PROGRAM MAIN

VAR CONSTANT
	// init pars for FB_CMA_SourcePaired, one dimensional signals with defined length
    cInitSourceVibration	: ST_MA_MultiArray_InitPars := (eTypeCode := eMA_TypeCode_LREAL, nDims := 1, aDimSizes := [cBufferLengthVib]);
	cInitSourcePosition		: ST_MA_MultiArray_InitPars := (eTypeCode := eMA_TypeCode_LREAL, nDims := 1, aDimSizes := [cBufferLengthPos]);	
END_VAR

VAR
	(* Properties of generated synthetic signals *)
	Amplitude			: ARRAY [0..9]  OF LREAL := [5, 8, 4, 7, 10, 9, 0, 0, 0, 0];
	Orders       		: ARRAY [0..9]  OF LREAL := [20, 50 , 90, 100, 120, 0, 0, 0, 0, 0];
	fbvib 				: FB_VibrationSource(Amplitude, Orders, cShaftPerimeter);
	aBufferVibration	: ARRAY[1..cOversamples] OF LREAL;  // vibration signal 
	aBufferPosition		: LREAL;                            // position signal
	
	(* Virtual axis control *)
	axis 				: AXIS_REF;
	fb_power 			: MC_POWER;
	fb_move 			: MC_MoveAbsolute;
	fb_reset 			: MC_Reset;
	
	(* axis control *)
	nstate 			: UDINT;
	nmovestate 		: UDINT;
	
	(* Sources and sinks *)
	fbSourceOrderSpec	: FB_CMA_SourcePaired :=(	stInitParsA := cInitSourceVibration, 
													stInitParsB := cInitSourcePosition,
													nOwnID := eID_SourcePaired, aDestIDs := [eID_OrderSpec], nResultBuffers := 4 );	// Initialize source buffers
	fbSourcePowerSpec	: FB_CMA_Source :=(	stInitPars := cInitSourceVibration, nOwnID := eID_Source, aDestIDs := [eID_PwrSpec], nResultBuffers := 4 );	// Initialize source buffers
	
	fbSinkOrderSpec		: FB_CMA_Sink := (nOwnID := eID_Sink_OrderSpec);
	fbSinkPowerSpec		: FB_CMA_Sink := (nOwnID := eID_Sink_PwrSpec);
	
	(* Spectrum results *)	
	aOrderSpecResult	: ARRAY[1..cFFTResult] OF LREAL;	// Copy of result
	aPowerSpecResult	: ARRAY[1..cFFTResult] OF LREAL;	// Copy of result
	
	(* Reset analysis chain *)
	bReset				: BOOL := FALSE;

	(* Helper *)
	i					: UDINT;
	{attribute 'BaseUnit' := '< AngularVelocity, 1, 0, None>'}
	fMotorspeed 			: LREAL;
	{attribute 'BaseUnit' := '< Angular, 1, 0, None>'}
	fMotorposition 		: LREAL;
	{attribute 'BaseUnit' := '< Angular, 1, 0, None>'}
	
	(* error monitoring *)
	fbErrHist			: FB_HRErrHist; // 
END_VAR

(* Axis control - Order spectrum specific code, see line 78ff*)
fb_power(Axis := axis);
fb_move(Axis := axis);
fb_reset(Axis := axis);
axis.ReadStatus();
CASE nstate OF 
	0: (* Reset axis *)
		fb_move.Execute := FALSE;
		fb_reset(Axis := axis, Execute := TRUE);
		fb_reset.Execute := TRUE;
		IF NOT fb_reset.Busy THEN
			nstate := 1;
		END_IF
		
	1:	(* Enable axis *)
		fb_reset.Execute := FALSE;
		fb_power.Enable := TRUE;
		fb_power.Enable_Positive := TRUE;
		fb_power.Enable_Negative := TRUE;
		IF axis.Status.ControlLoopClosed THEN
			nstate :=2;
		END_IF 
		
	2:	(* Run virtual axis *)	
		CASE nmovestate OF
			0:
				fb_reset.Execute := FALSE;;
				fb_move.Position := 10000;
				fb_move.Velocity := 20 *cShaftPerimeter;
				fb_move.BufferMode := MC_Buffered;
				fb_move.Execute := TRUE;
				IF fb_move.Done THEN
					fb_move.Execute := FALSE;
					nmovestate:= 1;
				END_IF
			
			1:
				fb_reset.Execute := FALSE;;
				fb_move.Position := 50000;
				fb_move.Velocity := 33 *cShaftPerimeter;
				fb_move.BufferMode := MC_BlendingNext;
				fb_move.Execute := TRUE;
				IF fb_move.Done THEN
					fb_move.Execute := FALSE;
					nmovestate:= 2;
				END_IF
			
			2:
				fb_reset.Execute := FALSE;;
				fb_move.Position := 80000;
				fb_move.Velocity := 10 * cShaftPerimeter;
				fb_move.BufferMode := MC_BlendingNext;
				fb_move.Execute := TRUE;
				IF fb_move.Done THEN
					fb_move.Execute := FALSE;
					nmovestate:= 3;
				END_IF
			
			3:
				fb_reset.Execute := FALSE;;
				fb_move.Position := 10000;
				fb_move.Velocity := 37 *cShaftPerimeter;
				fb_move.BufferMode := MC_BlendingNext;
				fb_move.Execute := TRUE;
				IF fb_move.Done THEN
					fb_move.Execute := FALSE;
					nmovestate:= 4;
				END_IF
			
			4:
				fb_reset.Execute := FALSE;;
				fb_move.Position := 0;
				fb_move.Velocity := 15 * cShaftPerimeter;
				fb_move.BufferMode := MC_BlendingNext;
				fb_move.Execute := TRUE;
				IF fb_move.Done THEN
					fb_move.Execute := FALSE;
					nmovestate:= 0;
				END_IF
		END_CASE
	
		(* Generate Data *)
		fMotorspeed    := axis.NcToPlc.ActVelo / cShaftPerimeter;
		fMotorposition := axis.NcToPlc.ActPos;
		
		FOR i := 1 TO cOversamples BY 1 DO
			// assuming constant speed for 10 samples vib signal generation 
			//fbvib.x := aBufferPosition + i * (fMotorposition - aBufferPosition)/ cOversamples;
			//fbvib();
			//aBufferVibration[i] := fbvib.vib;
			fbvib(x :=	aBufferPosition + i * (fMotorposition - aBufferPosition)/ cOversamples, vib => aBufferVibration[i] );
		END_FOR
		aBufferPosition := fMotorposition;
		
		(* Check input data *)
		IF ABS(fMotorspeed) >= cMinRPM / 60 AND ABS(fMotorspeed) <= cMaxRPM / 60 THEN
			IF bReset = TRUE THEN
				fbSourceOrderSpec.ResetAnalysisChain();
				fbSourcePowerSpec.ResetAnalysisChain();
				bReset := FALSE;
			END_IF
		
			(* Source data *)
			fbSourceOrderSpec.InputStd( pDataInA 		:= ADR(aBufferVibration),
										nDataInSizeA 	:= SIZEOF(aBufferVibration),
										nDimsDataInA	:= 1,
										pDataInB		:= ADR(aBufferPosition),
										nDataInSizeB	:= SIZEOF(aBufferPosition),
										nDimsDataInB	:= 1,
										eElementTypeA	:= E_MA_ElementTypeCode.eMA_TypeCode_LREAL,
										eElementTypeB	:= E_MA_ElementTypeCode.eMA_TypeCode_LREAL,
										nOptionPars		:= 0 );
			IF fbSourceOrderSpec.bError THEN
				fbErrHist.AddError(bErr:=TRUE, hrErrCode:=fbSourceOrderSpec.hrErrorCode, sErrSource:='MAIN.fbSourceOrderSpec'); // error monitoring
				// ToDo: if error
			END_IF
			
			fbSourcePowerSpec.Input1DStd( pDataIn 		:= ADR(aBufferVibration),
									nDataInSize 	:= SIZEOF(aBufferVibration),
									eElementType	:= E_MA_ElementTypeCode.eMA_TypeCode_LREAL,
									nOptionPars		:= 0 );
			IF fbSourcePowerSpec.bError THEN
				fbErrHist.AddError(bErr:=TRUE, hrErrCode:=fbSourcePowerSpec.hrErrorCode, sErrSource:='MAIN.fbSourcePowerSpec'); // error monitoring
				// ToDo: if error
			END_IF
		ELSE // i.e. invalid motorspeed
			bReset := TRUE;
		END_IF

		(* Push results to sink *)
		fbSinkOrderSpec.Output1D(	pDataOut 		:= ADR(aOrderSpecResult), 
									nDataOutSize 	:= SIZEOF(aOrderSpecResult), 
									eElementType 	:= eMA_TypeCode_LREAL, 
									nWorkDim		:= 0,
									nElements	:= cFFTResult,
									pStartIndex 	:= 0,
									nOptionPars		:= 0,
									bNewResult		=>  );
		IF fbSinkOrderSpec.bError THEN
			fbErrHist.AddError(bErr:=TRUE, hrErrCode:=fbSinkOrderSpec.hrErrorCode, sErrSource:='MAIN.fbSinkOrderSpec'); // error monitoring
			// ToDo: if error
		END_IF
	
		fbSinkPowerSpec.Output1D(	pDataOut 		:= ADR(aPowerSpecResult), 
									nDataOutSize 	:= SIZEOF(aPowerSpecResult), 
									eElementType 	:= eMA_TypeCode_LREAL, 
									nWorkDim 		:= 0,
									nElements	:= cFFTResult,
									pStartIndex 	:= 0,
									nOptionPars		:= 0,
									bNewResult		=>  );
		IF fbSinkPowerSpec.bError THEN
			fbErrHist.AddError(bErr:=TRUE, hrErrCode:=fbSinkOrderSpec.hrErrorCode, sErrSource:='MAIN.fbSinkOrderSpec'); // error monitoring
			// ToDo: if error
		END_IF
END_CASE

END_PROGRAM
